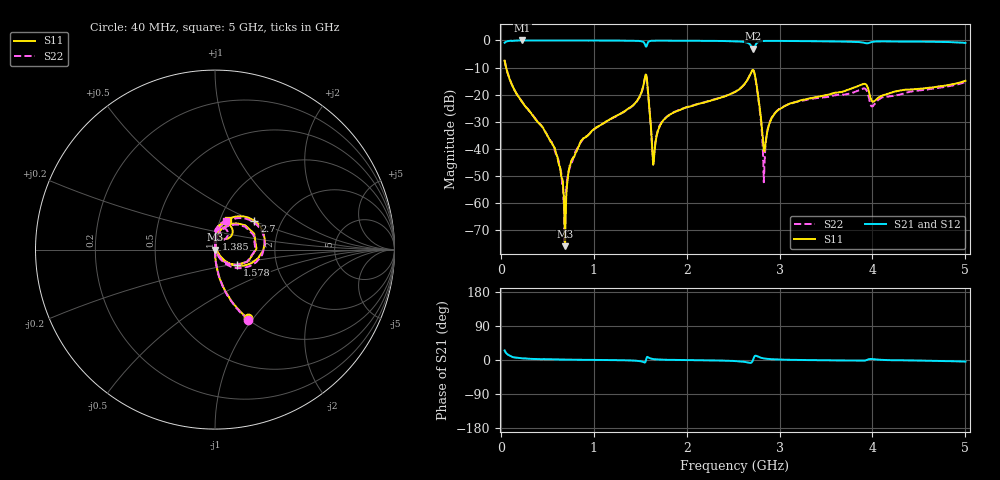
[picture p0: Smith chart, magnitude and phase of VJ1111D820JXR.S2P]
! VJ1111D820JXR
! DATE 02/16/2022  11:21
! CAPACITORS MOUNTED IN SERIES ON 25 MIL THICK MICROSTRIP SUBSTRATE
# GHz  S  MA  R  50.00
!  FREQ  S11M  S11A  S21M  S21A  S12M  S12A  S22M  S22A
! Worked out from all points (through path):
!   801 points, 40 MHz to 5 GHz, reference 50 ohm
!   highest |S21| = -0.01 dB at 232.2 MHz (marker M1); lowest = -3.0 dB at 2.718 GHz (marker M2)
!   lowest |S11| = -75.8 dB at 691 MHz (marker M3), VSWR 1.00, Z = 50 + j0.0162 ohm
!   |S11| at or under -10 dB: 56.34 MHz to end of sweep
!   |S22| runs from -74.0 to -7.3 dB; largest |S21 - S12| = 0.035
!   S11 on the Smith chart (normalised r, x): 40 MHz: 1.00, -0.94; 1.385 GHz: 1.00, +0.12; 1.578 GHz: 1.26, -0.22; 2.7 GHz: 1.46, +0.51; 5 GHz: 1.08, +0.37
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0.04  0.4239 -64.7  0.9058 25.1  0.9062 25.3  0.4319 -64.5
0.2322  0.07192 -86.3  0.9986 4.3  0.9975 4.9  0.07254 -86.1
0.567  0.0114 -88.7  0.9969 1.7  1.005 1.8  0.01116 -92.6
0.691  0.0001625 86.4  0.9969 1.0  1.004 0.8  0.0004291 35.4
0.7468  0.004998 91.4  0.9964 0.9  1.003 0.7  0.00481 81.0
0.8708  0.01449 88.4  0.9961 0.5  1.003 0.3  0.01411 87.2
1.3854  0.05745 84.9  0.9886 -1.1  0.9973 -1.3  0.05662 83.7
1.5466  0.1893 50.8  0.88 -6.7  0.8864 -6.9  0.1853 49.1
1.5776  0.1514 -34.6  0.8806 8.3  0.887 8.1  0.1469 -36.2
1.6396  0.005143 3.8  0.9889 2.5  0.9959 2.3  0.005424 12.7
1.6954  0.02279 87.2  0.9907 1.3  0.9991 1.1  0.02368 85.8
1.8566  0.04683 89.1  0.9898 0.2  0.9965 -0.0  0.04706 86.7
2.52  0.1124 80.9  0.9653 -2.8  0.974 -3.0  0.1127 78.8
2.6998  0.2725 36.3  0.7637 -6.3  0.7696 -6.4  0.2697 31.9
2.7184  0.2823 9.2  0.7059 2.9  0.7113 2.7  0.2782 4.2
2.8362  0.009123 24.0  0.978 4.0  0.985 3.8  0.004419 70.2
2.954  0.04644 88.5  0.9801 1.6  0.988 1.4  0.04697 92.5
3.3508  0.08773 86.9  0.9688 -0.3  0.9761 -0.6  0.08423 87.5
3.9026  0.1578 64.8  0.9108 -1.7  0.9179 -2.0  0.1302 68.9
4.0018  0.07421 57.6  0.9427 2.4  0.949 2.2  0.06096 71.9
4.1754  0.1053 81.8  0.9588 -0.4  0.9673 -0.6  0.09316 85.7
5  0.1806 67.2  0.8977 -4.2  0.9056 -4.5  0.1709 68.0
